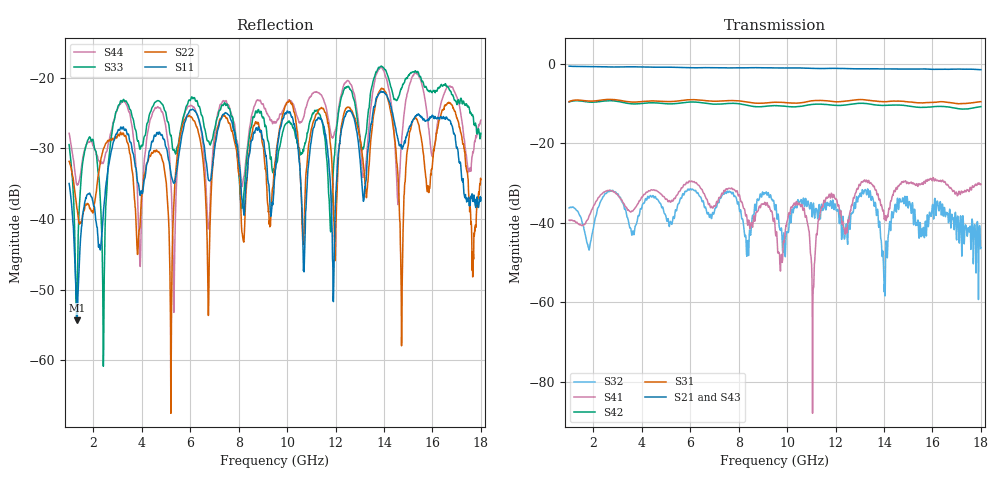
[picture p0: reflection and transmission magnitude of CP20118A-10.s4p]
! Amtery
! Email: info@amtery.com
! Phone: 886-2-2883-7839
! Model Number: CP20118A-10
! 4-port S-parameter measurement data for Bi-Directional Coupler
! Frequency Range: 1 GHz to 18 GHz
! Port 1: Input
! Port 2: Output
! Port 3: Coupled Forward
! Port 4: Coupled Reverse
# hz S db R 50
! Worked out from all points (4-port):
!   1361 points, 1 GHz to 18 GHz, reference 50 ohm
!   strongest paths, dB at 1 GHz, 5.25 GHz, 9.5 GHz, 13.75 GHz, 18 GHz:
!     S21: -0.7, -0.9, -1.1, -1.4, -1.5
!     S43: -0.7, -1.0, -1.3, -1.6, -1.7
!     S31: -9.6, -9.5, -9.7, -9.5, -9.6
!     S42: -9.7, -10.1, -10.6, -10.5, -10.8
!     S41: -39.4, -34.4, -41.0, -32.8, -30.3
!     S32: -36.3, -40.3, -36.8, -37.3, -46.4
!   lowest |S11| = -54.3 dB at 1.325 GHz (marker M1), VSWR 1.00, Z = 49.9 + j0.151 ohm
!   |S11| at or under -10 dB: start of sweep to end of sweep
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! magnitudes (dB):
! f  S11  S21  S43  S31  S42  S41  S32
! 1 GHz  -35.0  -0.7  -0.7  -9.6  -9.7  -39.4  -36.3
! 1.325 GHz  -54.3  -0.7  -0.8  -9.2  -9.3  -39.9  -37.0
! 3.188 GHz  -27.3  -0.8  -0.9  -9.4  -9.7  -34.5  -34.8
! 5.2 GHz  -33.6  -0.9  -1.0  -9.6  -10.1  -34.8  -39.9
! 5.825 GHz  -25.9  -1.0  -1.1  -9.2  -9.8  -30.1  -32.2
! 11.07 GHz  -27.2  -1.2  -1.4  -9.3  -10.3  -56.8  -35.5
! 18 GHz  -37.0  -1.5  -1.7  -9.6  -10.8  -30.3  -46.4
